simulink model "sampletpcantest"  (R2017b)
settings: Solver=FixedStepAuto  StartTime=0.0  StopTime=10.0  FixedStep=0.02  RelTol=1e-3  EnableMultiTasking=on
libraries: PCANLibrary x2

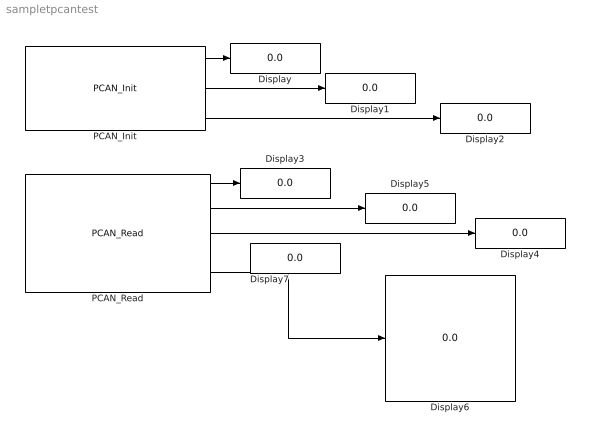
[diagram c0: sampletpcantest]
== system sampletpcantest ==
  Display{,1..7} (8 alike) : Display
  PCAN_Init : PCANLibrary/PCAN_Init  pcanusb=PCAN_USBBUS1  Initvar='1C'  MsgFormat=0  ToID='7FF'  FromID='00'
  PCAN_Read : PCANLibrary/PCAN_Read  PcanUsbChannel=PCAN_USBBUS1
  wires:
  PCAN_Init/1 -> Display/1
  PCAN_Init/2 -> Display1/1
  PCAN_Init/3 -> Display2/1
  PCAN_Read/1 -> Display3/1
  PCAN_Read/3 -> Display4/1
  PCAN_Read/2 -> Display5/1
  PCAN_Read/5 -> Display6/1
